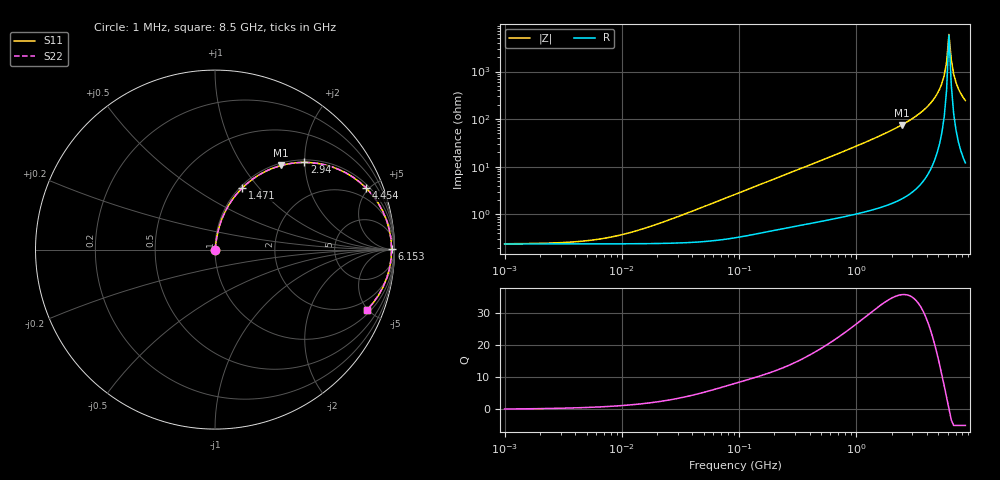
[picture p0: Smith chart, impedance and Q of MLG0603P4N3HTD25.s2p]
! S-Parameter Data Generated by TDK Corporation
! Copyright(C) 2025 TDK Corporation.
! All Rights Reserved.
! TDK P/N: MLG0603P4N3HTD25 (SMD / SMT Inductor (Coil))
! Property: L=4.3nH at 500MHz
! Size(LxWxT): 0.6x0.3x0.3mm
! Model Type: s2p (Touchstone File Format Version 1.0)
! Frequency: DC=Yes Start=1MHz Stop=8500MHz 198points Log-sweep
! Model Generated on Feb. 6, 2025
! Terms and conditions regarding TDK Simulation Models:
! 1)This simulation model is being provided solely for informational
!  purposes. Please refer to the specifications of the products in
!  terms of detailed characteristics of such products.
! 2)In no event shall TDK Corporation of any of its subsidiaries be
!  liable for any loss or damage arising, directly or indirectly,
!  from any information contained in this simulation model, including,
!  but not limited to loss or damages arising from any inaccuracies,
!  omissions or errors in connection with such information.
! 3)Any and all copyrights on this simulation model are owned by
!  TDK Corporation.  Duplication or redistribution of this simulation
!  model without prior written permission from TDK Corporation
!  is prohibited.
! 4)This simulation model is subject to any modification or change
!  without any prior notice.
! 5)Neither TDK Corporation nor any of its subsidiaries shall make any
!  warranty, express or implied, including but not limited to the
!  correctness, implied warranties of merchantability and fitness for
!  a particular purpose with respect to this simulation models.
! 6)The use of this simulation model shall be deemed to have consented
!  to the terms and conditions hereof.
! Port Assignments:
!  1 ---@@@--- 2
! Applicable Conditions:
!  Temperature = 25 degC
!  DC Bias Current = 0 A
!  Small Signal Operation
# Hz S MA R 50
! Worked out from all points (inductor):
!   197 points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, 1 MHz to 8.5 GHz, reference 50 ohm
!   read as one part in series: L = 4.56 nH near 26.51 MHz
!   highest Q = 35.8 at 2.444 GHz (marker M1), where L = 4.94 nH
!   self-resonance near 6.153 GHz
!   S11 on the Smith chart (normalised r, x): 1 MHz: 1.00, +0.00; 1.471 GHz: 1.03, +0.82; 2.94 GHz: 1.06, +1.99; 4.454 GHz: 1.21, +4.84; 6.153 GHz: open; 8.5 GHz: 1.24, -4.92
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1000000  0.002411 6.8  0.9976 -0.0  0.9976 -0.0  0.002411 6.8
4587603  0.002734 28.7  0.9976 -0.1  0.9976 -0.1  0.002734 28.7
9601846  0.003656 48.7  0.9976 -0.2  0.9976 -0.2  0.003656 48.7
2.10461e7  0.006507 67.6  0.9975 -0.3  0.9975 -0.3  0.006507 67.6
9.219544e7  0.02619 81.5  0.9965 -1.5  0.9965 -1.5  0.02619 81.5
4.229561e8  0.1132 80.2  0.9871 -6.5  0.9871 -6.5  0.1132 80.2
8.852465e8  0.2313 74.4  0.9637 -13.4  0.9637 -13.4  0.2313 74.4
1.470933e9  0.3757 66.1  0.9148 -22.1  0.9148 -22.1  0.3757 66.1
1.940355e9  0.486 59.3  0.86 -29.1  0.86 -29.1  0.486 59.3
2.444114e9  0.5965 51.8  0.7861 -36.6  0.7861 -36.6  0.5965 51.8
2.939772e9  0.6951 44.4  0.6994 -44.0  0.6994 -44.0  0.6951 44.4
3.703002e9  0.8214 33.0  0.5442 -55.2  0.5442 -55.2  0.8214 33.0
4.453958e9  0.9102 22.1  0.376 -65.4  0.376 -65.4  0.9102 22.1
5.115526e9  0.9583 13.0  0.2257 -72.9  0.2257 -72.9  0.9583 13.0
5.610304e9  0.9773 6.7  0.1173 -75.5  0.1173 -75.5  0.9773 6.7
5.87536e9  0.9823 3.5  0.06227 -71.7  0.06227 -71.7  0.9823 3.5
6.152938e9  0.984 0.2  0.01643 -12.9  0.01643 -12.9  0.984 0.2
6.44363e9  0.9825 -3.0  0.05518 70.0  0.05518 70.0  0.9825 -3.0
6.748056e9  0.9777 -6.3  0.1101 75.2  0.1101 75.2  0.9777 -6.3
7.066863e9  0.9699 -9.4  0.165 74.8  0.165 74.8  0.9699 -9.4
7.400733e9  0.9591 -12.6  0.2189 73.0  0.2189 73.0  0.9591 -12.6
8.5e9  0.911 -21.7  0.3702 65.5  0.3702 65.5  0.911 -21.7
